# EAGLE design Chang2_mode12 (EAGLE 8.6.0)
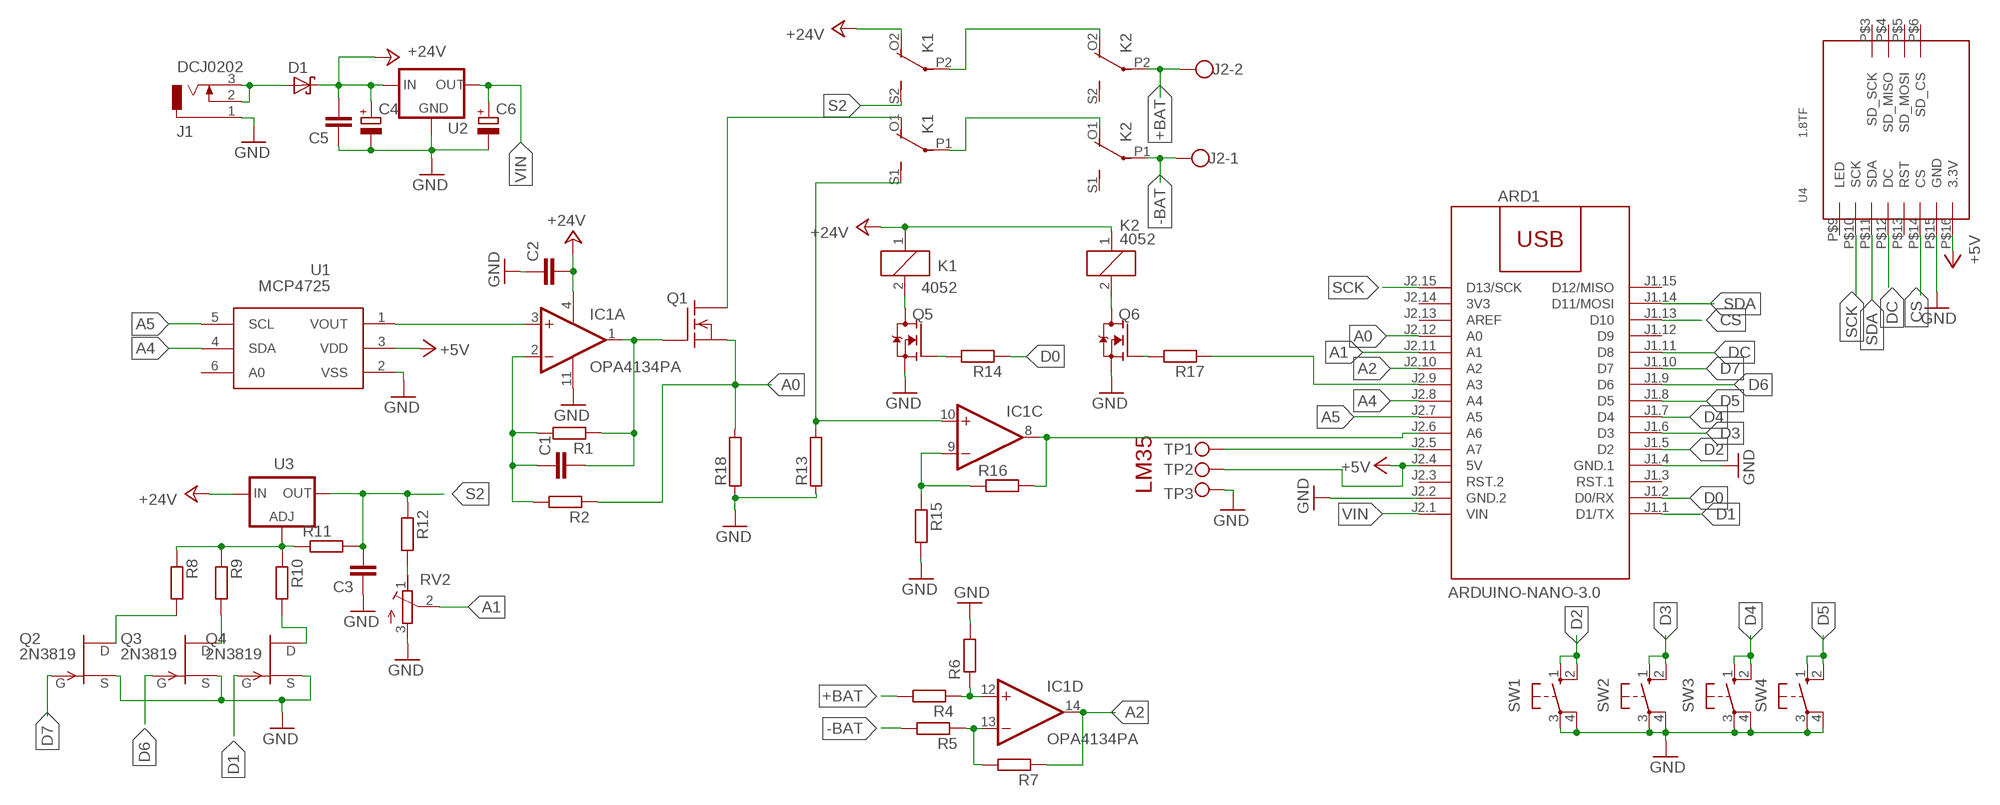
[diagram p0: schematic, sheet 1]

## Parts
ARD1  ARDUINO-NANO-3.0  [ARDUINO-NANO-3.0]
C1  C-EUC1206  [C1206]
C2  C-EUC1206  [C1206]
C3  C-EUC1206  [C1206]
C4  CPOL-EUSMCC  [SMC_C]
C5  C-EUC1206  [C1206]
C6  CPOL-EUSMCC  [SMC_C]
D1  MBRS320T3  [SMC]
IC1  OPA4134PA  [DIL14]
J1  DCJ0202  [DCJ0202]
J2  W237-102  [W237-102]
K1  4052  [F4052]
K2  4052  [F4052]
Q1  BUZ325V  [TO218V]
Q2  2N3819  [TO92]
Q3  2N3819  [TO92]
Q4  2N3819  [TO92]
Q5  NTF3055L108  [SOT223]
Q6  NTF3055L108  [SOT223]
R1  R-EU_R1206  [R1206]
R2  R-EU_R1206  [R1206]
R4  R-EU_R1206  [R1206]
R5  R-EU_R1206  [R1206]
R6  R-EU_R1206  [R1206]
R7  R-EU_R1206  [R1206]
R8  R-EU_R1206  [R1206]
R9  R-EU_R1206  [R1206]
R10  R-EU_R1206  [R1206]
R11  R-EU_R1206  [R1206]
R12  R-EU_R1206  [R1206]
R13  RAC05  [AC05]
R14  R-EU_R1206  [R1206]
R15  R-EU_R1206  [R1206]
R16  R-EU_R1206  [R1206]
R17  R-EU_R1206  [R1206]
R18  RAC05  [AC05]
RV2  R-TRIMM-3386-F  [R-TRIMM-3386F]
SW1  40-XX  [B3F-40XX]
SW2  40-XX  [B3F-40XX]
SW3  40-XX  [B3F-40XX]
SW4  40-XX  [B3F-40XX]
TP1  TPPAD1-13  [P1-13]
TP2  TPPAD1-13  [P1-13]
TP3  TPPAD1-13  [P1-13]
U1  MCP4725  [SOT23-6]
U2  78XXS  [78XXS]
U3  LM317MABT  [TO220L1]
U4  1.8TF  [1.8TFT]

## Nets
+5V: ARD1.J2.4(5V) TP2.TP U1.3(VDD) U4.P$16(3.3V)
+24V: C2.2 C4.+ C5.2 D1.C IC1.4(P:V+) K1.1 K1.O2(3:O) K2.1 U2.IN U3.3(IN)
+BAT: J2.2 K2.P2(3:P) R4.2
-BAT: J2.1 K2.P1(2:P) R5.2
A0: ARD1.J2.12(A0) Q1.3(S) R2.1 R18.2
A1: ARD1.J2.11(A1) RV2.2(S)
A2: ARD1.J2.10(A2) IC1.14(D:OUT) R7.1
A4: ARD1.J2.8(A4) U1.4(SDA)
A5: ARD1.J2.7(A5) U1.5(SCL)
CS: ARD1.J1.13(D10) U4.P$14(CS)
D0: ARD1.J1.2(D0/RX) R14.1
D1: ARD1.J1.1(D1/TX) Q4.2(G)
D2: ARD1.J1.5(D2) SW1.1(S) SW1.2(S1)
D3: ARD1.J1.6(D3) SW2.1(S) SW2.2(S1)
D4: ARD1.J1.7(D4) SW3.1(S) SW3.2(S1)
D5: ARD1.J1.8(D5) SW4.1(S) SW4.2(S1)
D6: ARD1.J1.9(D6) Q3.2(G)
D7: ARD1.J1.10(D7) Q2.2(G)
DC: ARD1.J1.11(D8) U4.P$12(DC)
GND: ARD1.J1.4(GND.1) ARD1.J2.2(GND.2) C2.1 C3.1 C4.- C5.1 C6.- IC1.11(P:V-) J1.1 Q2.3(S) Q3.3(S) Q4.3(S) Q5.3(S) Q6.3(S) R6.2 R13.1 R15.2 R18.1 RV2.3(E) SW1.3(P) SW1.4(P1) SW2.3(P) SW2.4(P1) SW3.3(P) SW3.4(P1) SW4.3(P) SW4.4(P1) TP3.TP U1.2(VSS) U2.GND U4.P$15(GND)
N$1: C1.2 IC1.1(A:OUT) Q1.1(G) R1.1
N$2: R8.1 R9.1 R10.1 R11.1 U3.1(ADJ)
N$4: IC1.3(A:+IN) U1.1(VOUT)
N$5: Q3.1(D) R9.2
N$6: C1.1 IC1.2(A:-IN) R1.2 R2.2
N$7: D1.A J1.2 J1.3
N$8: IC1.12(D:+IN) R4.1 R6.1
N$9: IC1.13(D:-IN) R5.1 R7.2
N$10: ARD1.J2.9(A3) R17.1
N$11: Q2.1(D) R8.2
N$12: ARD1.J2.5(A7) TP1.TP
N$13: Q4.1(D) R10.2
N$14: R12.2 RV2.1(A)
N$15: K1.2 Q5.2(D) Q5.4(D)
N$16: K1.O1(2:O) Q1.2(D)
N$17: IC1.10(C:+IN) K1.S1(2:S) R13.2
N$18: IC1.9(C:-IN) R15.1 R16.1
N$19: Q5.1(G) R14.2
N$20: ARD1.J2.6(A6) IC1.8(C:OUT) R16.2
N$21: K2.2 Q6.2(D) Q6.4(D)
N$22: K1.P2(3:P) K2.O2(3:O)
N$23: Q6.1(G) R17.2
N$24: K1.P1(2:P) K2.O1(2:O)
S2: C3.2 K1.S2(3:S) R11.2 R12.1 U3.2(OUT)
SCK: ARD1.J2.15(D13/SCK) U4.P$10(SCK)
SDA: ARD1.J1.14(D11/MOSI) U4.P$11(SDA)
VIN: ARD1.J2.1(VIN) C6.+ U2.OUT
Unconnected: ARD1.J1.3(RST.1) ARD1.J1.12(D9) ARD1.J1.15(D12/MISO) ARD1.J2.3(RST.2) ARD1.J2.13(AREF) IC1.5(B:+IN) IC1.6(B:-IN) IC1.7(B:OUT) K2.S1(2:S) K2.S2(3:S) U1.6(A0) U4.P$3(SD_SCK) U4.P$4(SD_MISO) U4.P$5(SD_MOSI) U4.P$6(SD_CS) U4.P$9(LED) U4.P$13(RST)

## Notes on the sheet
- LM35

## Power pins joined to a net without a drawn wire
3V3: ARD1.J2.14(3V3)

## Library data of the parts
ARD1 = diy-modules:ARDUINO-NANO-3.0: Arduino Nano 3.0 and compatible devices More details available here: https://www.arduino.cc/en/Main/ArduinoBoardNano Click here to find device on ebay.com
C1-C3 C5 = rcl:C-EU: CAPACITOR, European symbol
C4 C6 = rcl:CPOL-EU: POLARIZED CAPACITOR, European symbol
D1 = diode:MBRS3*0T3: SCHOTTKY BARRIER RECTIFIER 3.0 AMPERES 20, 30, 40 VOLT
IC1 = linear:OPA4*: Quad Operational Amplifier compatible with: TLC27L4 Low Power, Single-Supply, Rail-To-Rail Operational Amplifier Source: http://focus.ti.com/lit/ds/symlink/opa2345.pdf http://focus.ti.com .. opa241.pdf http://focus.ti.com .. tlc27l4.pdf http://focus.ti.com/lit/ds/symlink/opa2134.pdf
J1 = con-jack:DCJ0202: DC POWER JACK Source: DCJ0202.pdf; OC_FARNELL: unknown; OC_NEWARK: unknown
J2 = con-wago-500:W237-102: WAGO SCREW CLAMP; MPN: 237-102; OC_FARNELL: unknown; OC_NEWARK: 70K9898
K1 K2 = relay:4052: RELAY 2 x switch, Finder; OC_FARNELL: unknown; OC_NEWARK: unknown
Q1 = transistor-fet:BUZ325: N-Channel Enhancement MOSFET 400V; 10,5A; 0,5Ohm
Q2-Q4 = transistor-fet:2N3819: N-Channel Junction FET
Q5 Q6 = transistor-fet:NTF3055L108
R1 R2 R4-R12 R14-R17 = rcl:R-EU_: RESISTOR, European symbol
R13 R18 = resistor-power:R: Power Resitor; OC_FARNELL: unknown; OC_NEWARK: unknown
RV2 = rcl:R-TRIMM-3386-F
SW1-SW4 = switch-omron:40-XX: OMRON SWITCH; MF: OMRON COMPONENTS USA; MPN: B3F-4000; OC_FARNELL: 176434; OC_NEWARK: 36K3105
TP1-TP3 = testpad:TP: Test pad
U1 = linear:MCP4725
U2 = v-reg:78XXS: VOLTAGE REGULATOR
U3 = v-reg:LM317?*: 500 mA Adjustable Output Positive Voltage Regulator Source: http://www.onsemi.co.jp .. LM317M-D.PDF
U4 = tft_1_8_1_44_oled_0_96:1.8TF

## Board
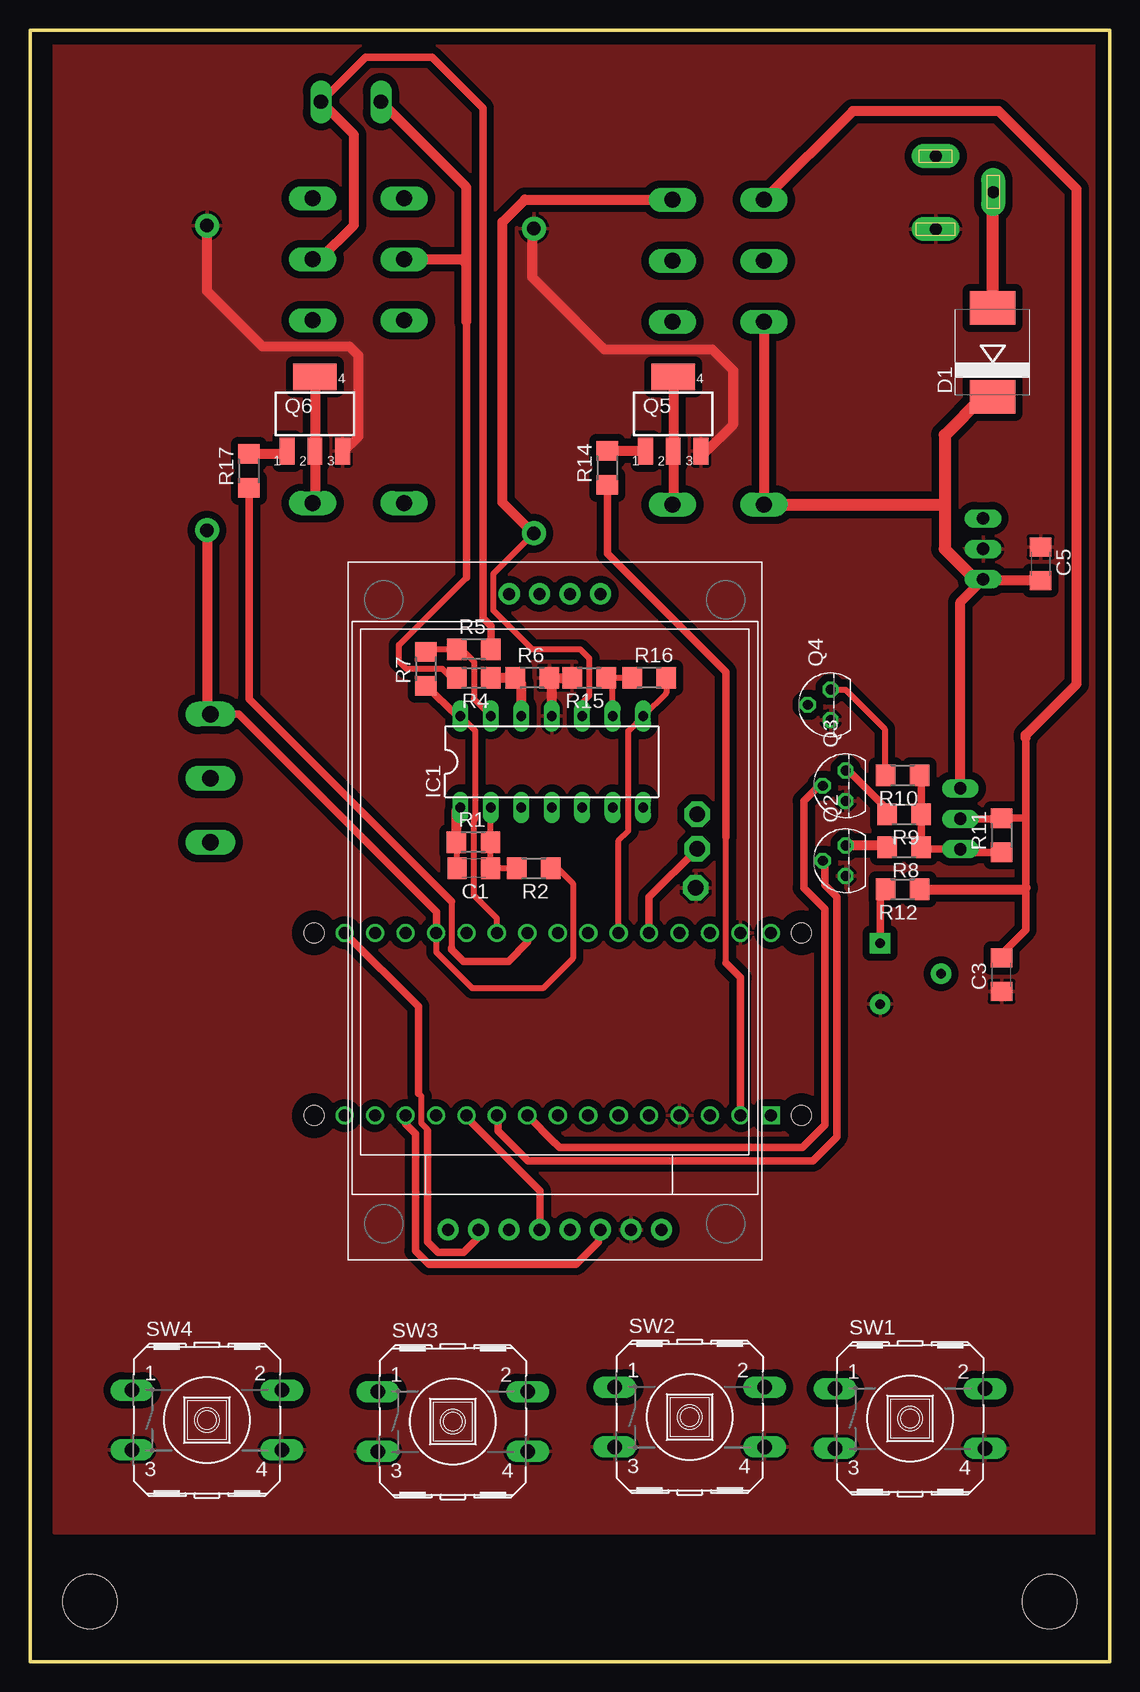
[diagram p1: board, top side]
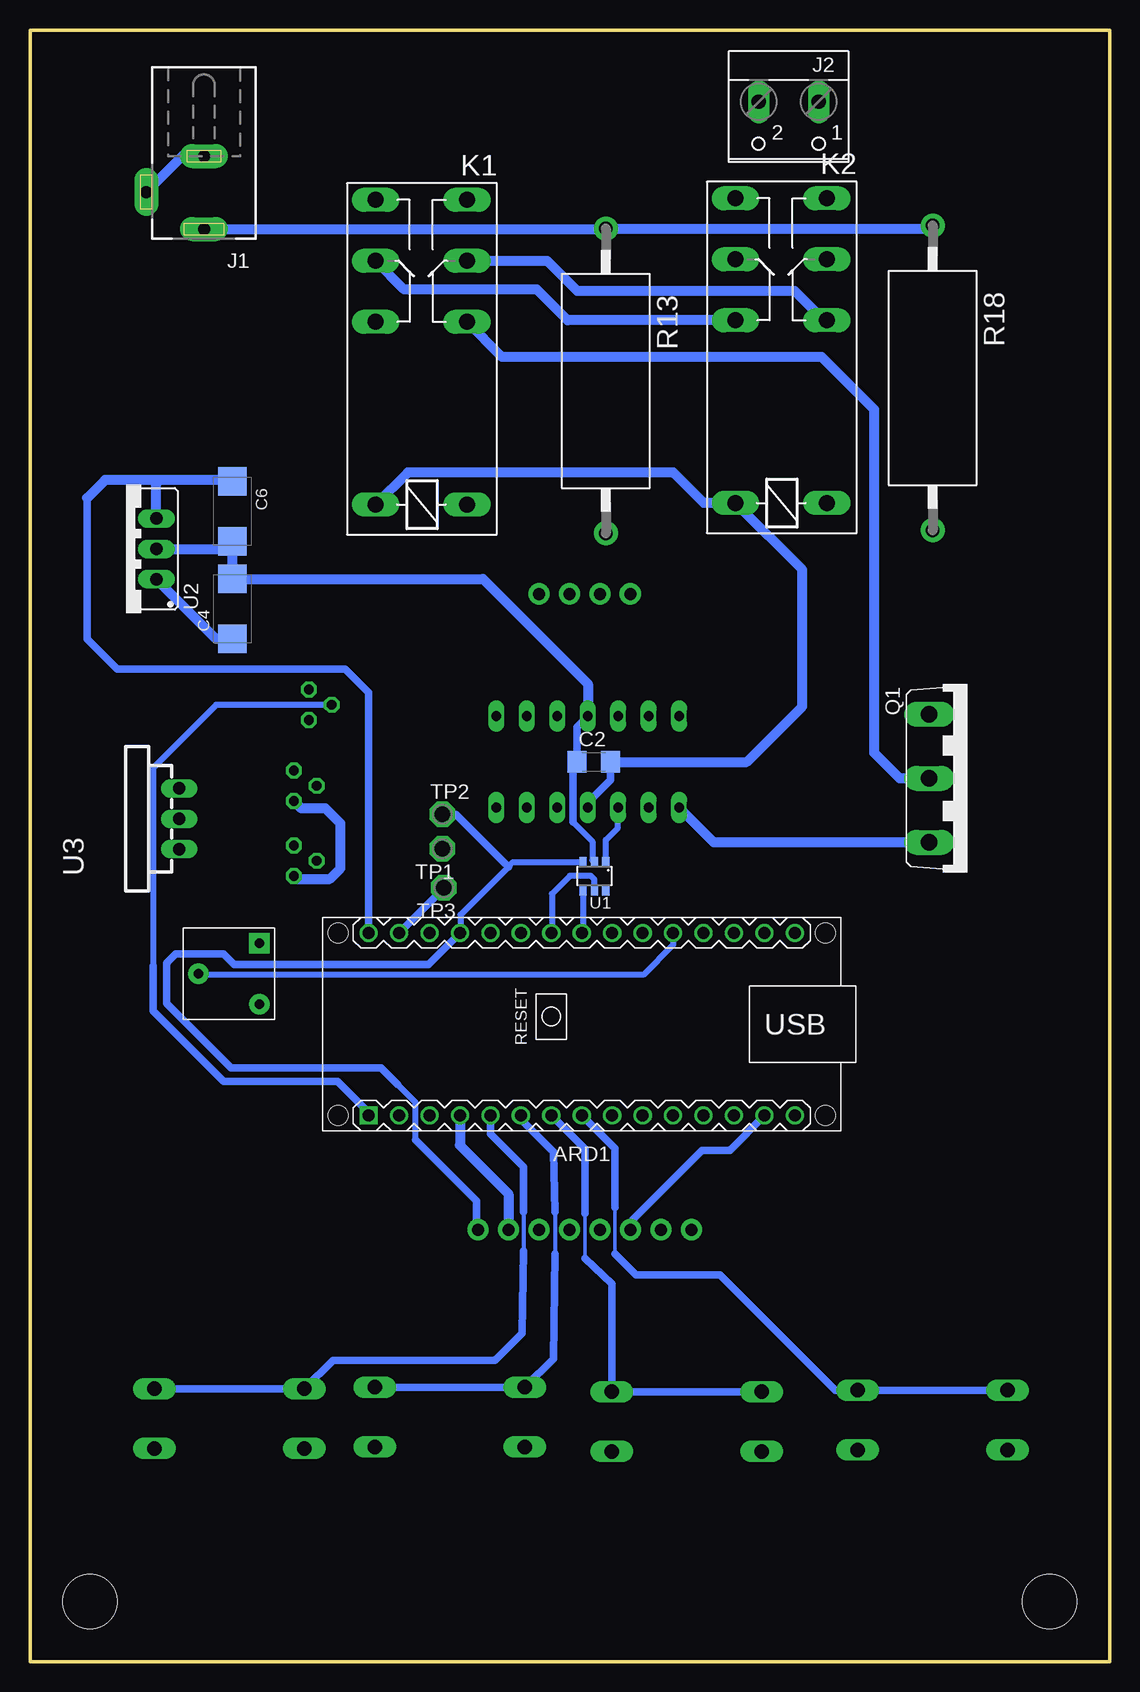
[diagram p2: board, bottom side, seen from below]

Size 90 x 136 mm. Coordinates in mm from the lower left corner, seen from the top.
Outline: 0,0 90,0 90,136 0,136 0,0
Copper layers (1*16): Top 0.035mm / dielectric 1.5mm / Bottom 0.035mm
Design rules "default *": minimum track width 10mil, minimum drill 24mil, track to track 8mil, track to pad 6mil, pad to pad 8mil, via to via 8mil, smd to smd 8mil, copper to edge 40mil, drill to drill 8mil, minimum pad ring 10mil, minimum via ring 8mil, stop-mask expansion 4mil, vias tented up to drill 0mil, thermal gap 10mil
Holes 4.5 mm at 5,5 85,5

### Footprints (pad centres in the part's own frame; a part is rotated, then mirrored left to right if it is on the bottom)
ARDUINO-NANO-3.0 = drill 1 square: J1.1 17.78,7.62 | drill 1: J1.2 15.24,7.62; J1.3 12.7,7.62; J1.4 10.16,7.62; J1.5 7.62,7.62; J1.6 5.08,7.62; J1.7 2.54,7.62; J1.8 0,7.62; J1.9 -2.54,7.62; J1.10 -5.08,7.62; J1.11 -7.62,7.62; J1.12 -10.16,7.62; J1.13 -12.7,7.62; J1.14 -15.24,7.62; J1.15 -17.78,7.62; J2.1 17.78,-7.62; J2.2 15.24,-7.62; J2.3 12.7,-7.62; J2.4 10.16,-7.62; J2.5 7.62,-7.62; J2.6 5.08,-7.62; J2.7 2.54,-7.62; J2.8 0,-7.62; J2.9 -2.54,-7.62; J2.10 -5.08,-7.62; J2.11 -7.62,-7.62; J2.12 -10.16,-7.62; J2.13 -12.7,-7.62; J2.14 -15.24,-7.62; J2.15 -17.78,-7.62 | hole 1.651: -20.32,7.62; -20.32,-7.62; 20.32,-7.62; 20.32,7.62
C1206 = smd 1.6 x 1.8: 1 -1.4,0; 2 1.4,0
SMC_C = smd 2.4 x 2.4: + -2.5,0; - 2.5,0
SMC = smd 2.8 x 3.8: A 3.7,0; C -3.7,0
DIL14 = drill 0.813 long: 1 -7.62,-3.81; 2 -5.08,-3.81; 3 -2.54,-3.81; 4 0,-3.81; 5 2.54,-3.81; 6 5.08,-3.81; 7 7.62,-3.81; 8 7.62,3.81; 9 5.08,3.81; 10 2.54,3.81; 11 0,3.81; 12 -2.54,3.81; 13 -5.08,3.81; 14 -7.62,3.81
DCJ0202 = drill 1 pad 2 long: 1 0,3.1; 2 4.8,0; 3 0,-3
W237-102 = drill 1.194 long: 1 -2.5,-1.27; 2 2.5,-1.27
F4052 = drill 1.321 long: 1 -3.81,3.81; 2 -3.81,-3.81; O1 11.43,-3.81; O2 11.43,3.81; P1 16.51,-3.81; P2 16.51,3.81; S1 21.59,-3.81; S2 21.59,3.81
TO218V = drill 1.397 long: 1 5.334,-3.175; 2 0,-3.175; 3 -5.334,-3.175
TO92 = drill 0.813 octagon: 1 1.27,0; 2 0,1.905; 3 -1.27,0
SOT223 = smd 1.219 x 2.235: 1 -2.311,-3.099; 2 0,-3.099; 3 2.311,-3.099 | smd 3.6 x 2.2: 4 0,3.099
R1206 = smd 1.6 x 1.803: 1 -1.422,0; 2 1.422,0
AC05 = drill 1.1 pad 2: 1 -12.7,0; 2 12.7,0
R-TRIMM-3386F = drill 0.8 pad 1.676 square: 1 0,0 | drill 0.8 pad 1.676: 2 5.08,2.54; 3 0,5.08
B3F-40XX = drill 1.194 long: 1 -6.248,2.489; 2 6.248,2.489; 3 -6.248,-2.489; 4 6.248,-2.489
P1-13 = drill 1.321 pad 2.159 octagon: TP 0,0
SOT23-6 = smd 0.6 x 0.9: 1 -0.95,-1.15; 2 0,-1.15; 3 0.95,-1.15; 4 0.95,1.15; 5 0,1.15; 6 -0.95,1.15
78XXS = drill 1.016 long: GND 0,-2.54; IN -2.54,-2.54; OUT 2.54,-2.54
TO220L1 = drill 1.016 long: 1 -2.54,-3.81; 2 0,-3.81; 3 2.54,-3.81
1.8TFT = drill 1 pad 1.778: P$3 55.5,21.05; P$4 55.5,18.52; P$5 55.5,15.98; P$6 55.5,13.44; P$9 2.5,26.14; P$10 2.5,23.6; P$11 2.5,21.06; P$12 2.5,18.52; P$13 2.5,15.98; P$14 2.5,13.44; P$15 2.5,10.9; P$16 2.5,8.36

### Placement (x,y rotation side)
ARD1  44,53.12 180 bottom
C1  37,66.12 180 top
C2  43,75 0 bottom
C3  81,57.25 90 top
C4  73.12,87.75 90 bottom
C5  84.25,91.5 270 top
C6  73.12,95.88 270 bottom
D1  80.25,109.12 90 top
IC1  43.5,75 0 top
J1  75.5,122.5 180 bottom
J2  26.75,128.75 180 bottom
K1  57.38,100.25 90 bottom
K2  27.38,100.38 90 bottom
Q1  11.88,73.62 270 bottom
Q2  68,66.75 90 top
Q3  68,73 90 top
Q4  66.75,79.75 90 top
Q5  53.62,104 0 top
Q6  23.75,104 0 top
R1  36.97,68.3 0 top
R2  42,66.12 180 top
R4  37,82 180 top
R5  37,84.38 0 top
R6  41.88,82 0 top
R7  33,82.75 90 top
R8  72.88,67.88 180 top
R9  72.88,70.62 180 top
R10  72.75,73.88 180 top
R11  81,68.88 90 top
R12  72.75,64.38 180 top
R13  42,106.75 270 bottom
R14  48.12,99.5 90 top
R15  46.62,82 180 top
R16  51.62,82 0 top
R17  18.25,99.25 90 top
R18  14.75,107 270 bottom
RV2  70.88,59.88 180 bottom
SW1  73.38,20.25 0 top
SW2  55,20.38 0 top
SW3  35.25,20 0 top
SW4  14.75,20.12 0 top
TP1  55.62,67.75 180 bottom
TP2  55.62,70.62 0 bottom
TP3  55.5,64.5 180 bottom
U1  42.95,65.47 180 bottom
U2  82,92.75 90 bottom
U3  81.38,70.25 90 bottom
U4  61,33.5 90 top

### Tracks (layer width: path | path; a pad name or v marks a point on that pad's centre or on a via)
+5V
  Bottom 0.5: U1.3 49.76,66.62 50.12,66.25 54.12,62.25 54.12,60.78 ARD1.J2.4 | 57.88,43.5 57.88,46.62 59.38,48.12
  Bottom 0.61: 57.88,43.5 52.76,38.38 52.76,36.12 U4.P$16 | 59.38,48.12 60.75,49.5 73.25,49.5 78.62,54.88 78.62,58.25 77.88,59 73.88,59 73,58.12 56.78,58.12 ARD1.J2.4 | TP2.TP 54.5,70.62 50.12,66.25
+24V
  Top 0.813: K1.O2 K1.1 | U3.3 77.56,88.31 U2.IN 79.57,90.1 C5.2
  Top 1.016: D1.C 79.42,105.42 76.25,102.25 76.25,96.25 | 76.25,96.25 76.25,92.75 78.75,90.25 79.42,90.25 U2.IN | K1.1 76.06,96.44 76.25,96.25
  Bottom 0.61: IC1.4 43.5,71.62 41.62,73.5 41.62,74.97 C2.2
  Bottom 0.813: K1.1 58.5,99.12 36.38,99.12 33.81,96.56 K2.1 25.62,91 25.62,79.62 30.25,75 C2.2 | C4.+ 74.5,85.25 U2.IN
+BAT
  Top 0.5: R4.2 35.12,82 34.38,82.75 31.38,82.75 30.75,83.38 30.75,84.75 36.38,90.38
  Top 0.61: 36.38,90.38 36.38,111.69
  Top 0.813: 36.38,111.69 36.38,116.5 | 36.38,116.5 36.38,122.89 J2.2 | K2.P2 35.99,116.89 36.38,116.5
-BAT
  Top 0.61: R5.2 38.42,86.33 37.75,87 37.75,129.5 33.5,133.75 27.98,133.75 J2.1
  Top 0.813: K2.P1 24.14,116.89 27,119.75 27,127.27 J2.1
A0
  Top 0.5: R2.1 44,66.12 45.25,64.88 45.25,58.62 42.75,56.12 36.88,56.12 33.88,59.12 33.88,60.71 ARD1.J2.12
  Top 0.61: Q1.3 17.42,78.96 33.88,62.5 33.88,60.78 ARD1.J2.12
  Top 0.813: R18.2 14.75,79.26 Q1.3
A1
  Bottom 0.5: ARD1.J2.11 36.38,59.74 38.88,57.25 75.87,57.25 RV2.2
A2
  Top 0.5: ARD1.J2.10 38.92,61.95 37,63.88 37,70.12 37.12,70.25 37.12,77.56 IC1.14
  Top 0.61: IC1.14 35.64,78.81 R7.1
A4
  Bottom 0.5: U1.4 43.9,60.84 ARD1.J2.8
A5
  Bottom 0.5: U1.5 42.95,65.2 43.25,65.5 45,65.5 46.5,64 46.5,60.78 ARD1.J2.7
CS
  Top 0.61: ARD1.J1.13 31.3,44.83 32.12,44 32.12,34.25 33.25,33.12 45.5,33.12 47.38,35 47.38,35.81 U4.P$14
D0
  Top 0.5: 58,58.25 58,68.75
  Top 0.61: R14.1 48.12,92.38 58,82.5 58,68.75 | ARD1.J1.2 59.24,57.01 58,58.25
D1
  Bottom 0.5: Q4.2 74.5,79.75 79.75,74.5 79.75,58
  Bottom 0.61: 79.75,58 79.75,54.25 73.88,48.38 64.38,48.38 61.78,45.78 ARD1.J1.1
D2
  Bottom 0.35: 48.88,37.5 48.88,34.25
  Bottom 0.61: SW1.2 SW1.1 64.74,25.12 51.25,25.12 49,27.38 48.88,34.25 | ARD1.J1.5 51.62,43.99 48.88,41.25 48.88,37.5
D3
  Bottom 0.35: 46.25,37.5 46.25,34
  Bottom 0.61: SW2.2 SW2.1 46.38,25.24 46.25,34 | ARD1.J1.6 49.08,45.2 46.38,42.5 46.25,37.5
D4
  Bottom 0.3: 43.75,33.62 43.75,37.38
  Bottom 0.61: 43.75,33.62 41.5,31.5 SW3.2 SW3.1 | ARD1.J1.7 43.75,42.72 43.75,37.38
D5
  Bottom 0.3: 41.25,34 41.25,37.88
  Bottom 0.61: 41.25,34 39.5,32.25 32.5,32.25 22.86,22.61 SW4.2 SW4.1 | ARD1.J1.8 41.25,42.76 41.25,37.88
D6
  Top 0.61: Q3.2 65.75,73 64.5,71.75 64.5,64.5 66.25,62.75 66.25,44.75 64.38,42.88 44.12,42.88 43.75,43.25 43.72,43.25 ARD1.J1.9
D7
  Top 0.61: ARD1.J1.10 39,45.42 39,44.25 41.5,41.75 65.25,41.75 67.25,43.75 67.25,63.75 66.25,64.75 66.25,66.59 Q2.2
DC
  Top 0.61: ARD1.J1.11 36.38,45.37 42.5,39.25 42.5,36.02 U4.P$12
GND
  Top 0.813: IC1.11 43.5,81.8 R6.2 R15.2 | Q6.3 26.15,100.9 27.38,102.12 27.38,108.88 26.62,109.62 19.38,109.62 14.75,114.25 R18.1 | Q5.3 56.4,100.9 58.62,103.12 58.62,107.62 56.88,109.38 47.88,109.38 41.88,115.38 41.88,119.33 R13.1
  Bottom 0.406: 50.12,36.02 50.1,36.02 U4.P$15
  Bottom 0.5: 44.75,70 43.12,68.38 43.12,66.8 U1.2
  Bottom 0.61: 44.75,70 44.75,74.65 C2.1 44.4,77.91 IC1.11 | TP3.TP 55.5,64.48 ARD1.J2.2
  Bottom 0.813: R18.1 15,119.45 R13.1 42.05,119.4 J1.1 | 43.25,79.06 IC1.11 43.5,81.5 52.25,90.25 C4.- C6.- 73.75,92.75 U2.GND | ARD1.J1.4 54.16,43.03 50.12,39 50.12,36.02 | Q2.3 67.98,65.48 67.75,65.25 65,65.25 64.12,66.12 64.12,69.88 65.38,71.12 67.39,71.12 Q3.3
  pour Top (isolate 0.61): 2,135 89.5,135 89.5,10.75 2,10.75
N$1
  Top 0.5: C1.2 35.6,68.24 R1.1
  Top 0.813: R1.1 35.55,70.86 IC1.1
  Bottom 0.813: Q1.1 32.98,68.29 IC1.1
N$2
  Top 0.61: R10.1 74.3,73.75 R9.1 R8.1 74.46,67.71 U3.1 77.82,67.45 R11.1
N$4
  Bottom 0.5: U1.1 42,68.5 41,69.5 41,71.15 IC1.3
N$5
  Top 0.61: R9.2 71.45,71.05 68.5,74 68.27,74 Q3.1
N$6
  Top 0.5: R2.2 C1.1 38.4,68.29 R1.2 38.39,71.16 IC1.2
N$7
  Top 1.016: D1.A 80.25,122.45 J1.2
  Bottom 0.813: J1.3 77.3,125.5 J1.2
N$8
  Top 0.813: R4.1 R6.1 40.96,81.49 IC1.12
N$9
  Top 0.5: IC1.13 37,80.23 37,83.38 36,84.38 R5.1 33.2,84.38 R7.2
  Top 0.61: 33.2,84.25 R7.2
N$10
  Top 0.5: 35.12,63.38 35.12,59.5
  Top 0.61: R17.1 18.25,80.25 35.12,63.38 | 35.12,59.5 35.12,59.38 36.12,58.38 39.88,58.38 41.46,59.96 ARD1.J2.9
N$11
  Top 0.5: 71.31,68.02 R8.2
  Top 0.813: 71.31,68.02 Q2.1
N$12
  Top 0.61: ARD1.J2.5 51.62,63.74 TP1.TP
N$13
  Top 0.5: Q4.1 67.98,81.02 71.25,77.75 71.25,73.95 R10.2
N$14
  Top 0.61: RV2.1 70.88,63.92 R12.2
N$15
  Top 0.813: Q5.4 Q5.2 53.62,96.5 K1.2
N$16
  Bottom 0.813: Q1.2 17.5,73.62 19.62,75.75 19.62,104.38 24,108.75 50.63,108.75 K1.O1
N$17
  Top 0.5: IC1.10 46.04,79.92 46.62,80.5 46.62,83.62 45.88,84.38 41.88,84.38 38.62,87.62 38.62,90.67 R13.2
  Top 0.813: R13.2 41.95,94.05 39.38,96.62 39.38,120 41.25,121.88 53.53,121.88 K1.S1
N$18
  Top 0.5: IC1.9 48.58,81.47 48.4,81.65 | 48.4,81.65 R15.1 | R16.1 48.75,82 48.4,81.65
N$19
  Top 0.813: R14.2 51.29,100.92 Q5.1
N$20
  Top 0.5: ARD1.J2.6 49.08,68.45 49.88,69.25 49.88,77.56 IC1.8 53.05,80.74 R16.2
N$21
  Top 0.813: Q6.4 Q6.2 23.75,96.75 K2.2
N$22
  Bottom 0.813: K2.O2 45.18,111.81 47.75,114.38 58.8,114.38 K1.P2
N$23
  Top 0.813: R17.2 21.21,100.67 Q6.1
N$24
  Bottom 0.813: K2.O1 23.8,111.81 26.25,114.25 44.38,114.25 46.88,116.75 53,116.75 53.12,116.88 53.45,116.88 K1.P1
S2
  Top 0.61: U3.2 80.95,70.25 R11.2 82.95,70.3 83,70.25 | C3.2 81,59 83,61 83,64.5 83,70.25 | 83,70.25 83,77
  Top 0.813: R12.1 82.88,64.38 83,64.5 | 83,77 83,77.25 87.25,81.5 87.25,122.75 80.75,129.25 68.59,129.25 K1.S2
SCK
  Top 0.5: 33.12,44.25 33.12,44.38 32.62,44.88 32.62,47.12 32.38,47.38
  Top 0.61: 33.12,44.25 33.12,35 34,34.12 36.12,34.12 37.25,35.25 37.25,35.85 U4.P$10 | 32.38,47.38 32.38,54.59 ARD1.J2.15
SDA
  Bottom 0.61: ARD1.J1.14 31.64,42.62 34,42.62 39.75,36.88 39.75,36.19 U4.P$11
VIN
  Bottom 0.61: ARD1.J2.1 61.78,80.78 63.75,82.75 82.75,82.75 85.25,85.25 85.25,97
  Bottom 0.813: C6.+ 73.25,98.5 79.25,98.5 | 79.25,98.5 83.75,98.5 85.25,97 | U2.OUT 79.46,98.29 79.25,98.5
